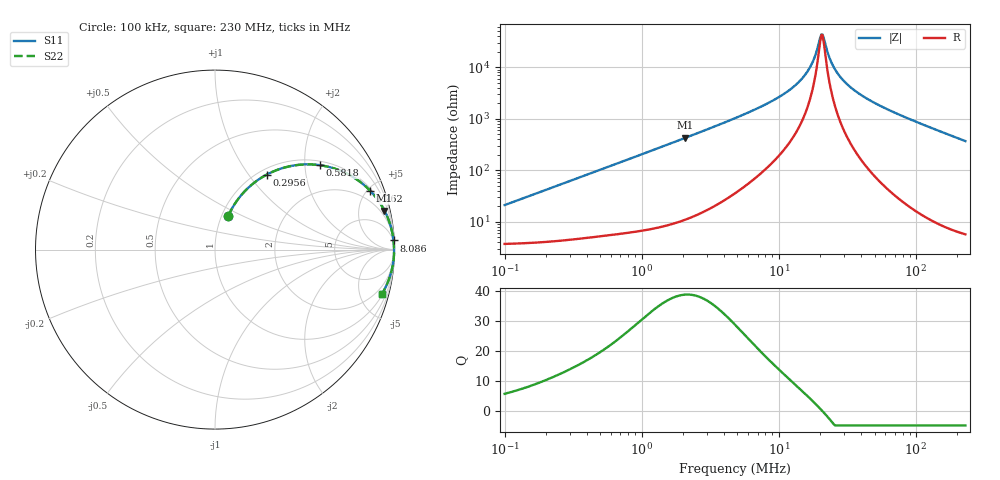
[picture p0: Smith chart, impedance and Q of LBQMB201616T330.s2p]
! LBQMB201616T330  S-PARAMETER MODEL  ( General Type )
! Model Generated by TAIYO YUDEN Corporation (http://www.ty-top.com)
! Version 1.0
! TAIYO YUDEN Control No. 191025NI43SB-FBB
! Copyright(c) 2019 TAIYO YUDEN CO.,LTD. All Rights Reserved.
! Product Description (link to TY-COMPAS)
! https://ds.yuden.co.jp/TYCOMPAS/or/detail?pn=LBQMB201616T330J&u=M
! Products Name : Inductors
! Characteristics :
!  Inductance : 33 uH , SRF(min) : 15 MHz , DC Resistance(max) : 4.68 Ohm , Rated Current : 125 mA
!  Case Size : 2.0 x 1.6 / 0.079 x 0.063 [mm/inch] , Thickness : 1.6 / 0.063 [mm/inch]
!  (Conditions: Temperature = 25 degC , DC Bias Current/Voltage = 0A / 0V)
! External Node Assignments :
!  1  o---GGG---o  2
! GND o---------o GND
! Frequency Range : 0.1MHz  -  229.966873MHz  [ 402 STEP ]
# MHz S RI R 50
! Freq[MHz].  S11 Real  S11 Imag  S21 Real  S21 Imag  S12 Real  S12 Imag  S22 Real  S22 Imag
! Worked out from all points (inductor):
!   401 points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, 100 kHz to 230 MHz, reference 50 ohm
!   read as one part in series: L = 33.3 uH near 103.9 kHz
!   highest Q = 38.8 at 2.087 MHz (marker M1), where L = 32.8 uH
!   self-resonance near 20.47 MHz
!   S11 on the Smith chart (normalised r, x): 100 kHz: 1.07, +0.42; 295.6 kHz: 1.09, +1.23; 581.8 kHz: 1.11, +2.40; 1.262 MHz: 1.15, +5.18; 8.086 MHz: 3, +39; 230 MHz: 1.11, -7.42
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0.1  0.0738 0.1869  0.9262 -0.1869  0.9262 -0.1869  0.0738 0.1869
0.1787  0.1481 0.3055  0.8519 -0.3055  0.8519 -0.3055  0.1481 0.3055
0.295551  0.2886 0.418  0.7114 -0.418  0.7114 -0.418  0.2886 0.418
0.365661  0.3733 0.4532  0.6267 -0.4532  0.6267 -0.4532  0.3733 0.4532
0.581807  0.5863 0.47  0.4137 -0.47  0.4137 -0.47  0.5863 0.47
1.261669  0.8633 0.3293  0.1367 -0.3293  0.1367 -0.3293  0.8633 0.3293
1.337081  0.8761 0.3155  0.1239 -0.3155  0.1239 -0.3155  0.8761 0.3155
2.086669  0.9438 0.2178  0.0562 -0.2178  0.0562 -0.2178  0.9438 0.2178
4.889189  0.9879 0.0932  0.0121 -0.0932  0.0121 -0.0932  0.9879 0.0932
8.086211  0.9945 0.051  0.00548 -0.051  0.00548 -0.051  0.9945 0.051
10.80955  0.9962 0.0329  0.00376 -0.0329  0.00376 -0.0329  0.9962 0.0329
13.37375  0.997 0.0213  0.00299 -0.0213  0.00299 -0.0213  0.997 0.0213
15.61301  0.9974 0.0135  0.00262 -0.0135  0.00262 -0.0135  0.9974 0.0135
17.53523  0.9976 0.00783  0.00242 -0.00783  0.00242 -0.00783  0.9976 0.00783
20.07894  0.9977 0.00133  0.00226 -0.00133  0.00226 -0.00133  0.9977 0.00133
20.87128  0.9978 -0.000519  0.00223 0.000519  0.00223 0.000519  0.9978 -0.000519
24.36589  0.9978 -0.00798  0.0022 0.00798  0.0022 0.00798  0.9978 -0.00798
26.32686  0.9978 -0.0118  0.00222 0.0118  0.00222 0.0118  0.9978 -0.0118
29.56814  0.9977 -0.0176  0.00233 0.0176  0.00233 0.0176  0.9977 -0.0176
40.29866  0.9969 -0.0347  0.00309 0.0347  0.00309 0.0347  0.9969 -0.0347
64.11956  0.9936 -0.0671  0.00638 0.0671  0.00638 0.0671  0.9936 -0.0671
229.9669  0.929 -0.2492  0.071 0.2492  0.071 0.2492  0.929 -0.2492
